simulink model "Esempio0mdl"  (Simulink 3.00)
settings: Solver=ode45  StartTime=0.0  StopTime=1.0  RelTol=1e-3
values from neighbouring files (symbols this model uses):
  A = evalfr(gz,exp(T*wa*j))    [Formule_di_Inversione_discrete.m]    (also in Esempio0.m = 0.01; Controllo_CC_K.m = evalfr(Gz,exp(T*wa*j)))
  b = k*(T-2*tau1)    (= -1.462)    [Formule_di_Inversione_discrete.m]    (also in Esempio0.m = 0.1; Controllo_CC_K.m = 0.008; motore_CC_ES1.m = 0.8)
  Cm = 0.001    [Esempio0.m]
  Km = 10    [Esempio0.m]
  Kv = 1    [Esempio0.m]
  mp = 1    [Esempio0.m]
undefined symbols (not defined in the file or in its folder): Pmax
libraries: cstblocks x2

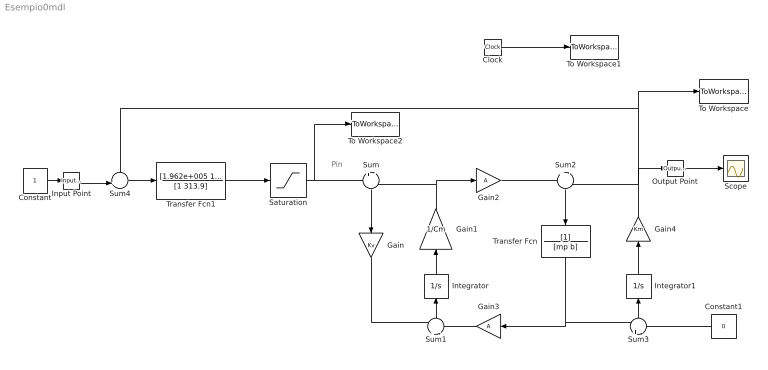
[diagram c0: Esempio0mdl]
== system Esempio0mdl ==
  note: Pin
  Clock : Clock
  Constant : Constant  Value=1
  Constant1 : Constant  Orientation=left  Value=0
  Gain : Gain  Orientation=down  Gain=Kv  SaturateOnIntegerOverflow=on
  Gain1 : Gain  Orientation=up  Gain=1/Cm  SaturateOnIntegerOverflow=on
  Gain2 : Gain  Gain=A  SaturateOnIntegerOverflow=on
  Gain3 : Gain  Orientation=left  Gain=A  SaturateOnIntegerOverflow=on
  Gain4 : Gain  Orientation=up  Gain=Km  SaturateOnIntegerOverflow=on
  Input Point : cstblocks/Input Point  PerturbationValue=0
  Integrator : Integrator  Orientation=up  ExternalReset=none  InitialConditionSource=internal  InitialCondition=0  LimitOutput=off  UpperSaturationLimit=inf  LowerSaturationLimit=-inf  ShowSaturationPort=off  ShowStatePort=off  AbsoluteTolerance=auto
  Integrator1 : Integrator  Orientation=up  ExternalReset=none  InitialConditionSource=internal  InitialCondition=0  LimitOutput=off  UpperSaturationLimit=inf  LowerSaturationLimit=-inf  ShowSaturationPort=off  ShowStatePort=off  AbsoluteTolerance=auto
  Output Point : cstblocks/Output Point  SigprobeOutputIndex=1
  Saturation : Saturate  UpperLimit=Pmax  LowerLimit=-Pmax
  Scope : Scope
  Sum : Sum  Orientation=down  Inputs=+|-  SaturateOnIntegerOverflow=on
  Sum1 : Sum  Orientation=up  Inputs=+|-  SaturateOnIntegerOverflow=on
  Sum2 : Sum  Orientation=down  Inputs=+|-  SaturateOnIntegerOverflow=on
  Sum3 : Sum  Orientation=up  Inputs=+|-  SaturateOnIntegerOverflow=on
  Sum4 : Sum  Inputs=-+|  SaturateOnIntegerOverflow=on
  To Workspace : ToWorkspace  VariableName=Fm  SampleTime=-1  SaveFormat=Matrix
  To Workspace1 : ToWorkspace  VariableName=t  SampleTime=-1  SaveFormat=Matrix
  To Workspace2 : ToWorkspace  VariableName=Pin  SampleTime=-1  SaveFormat=Matrix
  Transfer Fcn : TransferFcn  Orientation=down  Numerator=[1]  Denominator=[mp b]
  Transfer Fcn1 : TransferFcn  Numerator=[1.962e+005 1.962e+005*16.65]  Denominator=[1 313.9]
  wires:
  Constant/1 -> Input Point/1
  Input Point/1 -> Sum4/2
  Sum4/1 -> Transfer Fcn1/1
  Sum/1 -> Gain/1
  Gain/1 -> Sum1/1
  Sum1/1 -> Integrator/1
  Integrator/1 -> Gain1/1
  Gain1/1 -> Sum/2, Gain2/1
  Gain3/1 -> Sum1/2
  Gain2/1 -> Sum2/1
  Sum2/1 -> Transfer Fcn/1
  Integrator1/1 -> Gain4/1
  Sum3/1 -> Integrator1/1
  Transfer Fcn/1 -> Gain3/1, Sum3/1
  Constant1/1 -> Sum3/2
  Gain4/1 -> Sum2/2, Output Point/1, Sum4/1, To Workspace/1
  Output Point/1 -> Scope/1
  Clock/1 -> To Workspace1/1
  Transfer Fcn1/1 -> Saturation/1
  Saturation/1 -> Sum/1, To Workspace2/1
